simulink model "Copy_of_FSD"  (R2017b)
settings: Solver=FixedStepDiscrete  StartTime=0.0  StopTime=10.0  FixedStep=0.01  RelTol=1e-3  EnableMultiTasking=on
undefined symbols (not defined in the file): ASWTYPE_FALSE, ASWTYPE_TRUE, CcFSD_MSDOpenFltDelTi_ms, CcFSD_MSDOpenPackVolt_V, CcFSD_MSDOpenSumCellVolt_V, FSD_RUNTIME_MS
libraries: AIWAYS_Powertrain_BMS_lib x6

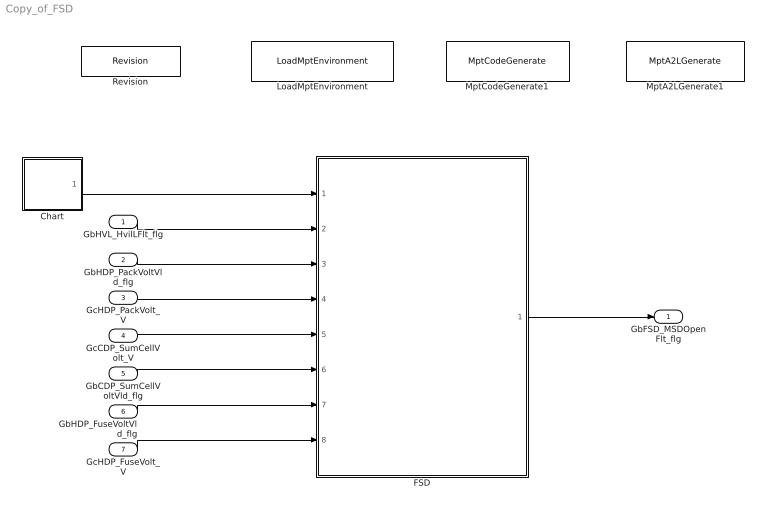
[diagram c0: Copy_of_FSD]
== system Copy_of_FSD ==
  GbHVL_HvilLFlt_flg : Inport
  GbHDP_PackVoltVld_flg : Inport  Port=2
  GcHDP_PackVolt_V : Inport  Port=3
  GcCDP_SumCellVolt_V : Inport  Port=4
  GbCDP_SumCellVoltVld_flg : Inport  Port=5
  GbHDP_FuseVoltVld_flg : Inport  Port=6
  GcHDP_FuseVolt_V : Inport  Port=7
  Chart : Stateflow chart  TreatAsAtomicUnit=on
  FSD : Subsystem
  LoadMptEnvironment : AIWAYS_Powertrain_BMS_lib/Config/LoadMptEnvironment  ProjectName=Comm  SuppierID=NewPlatformUAES
  MptA2LGenerate1 : AIWAYS_Powertrain_BMS_lib/Config/MptA2LGenerate  SystemSampleTime=-1
  MptCodeGenerate1 : AIWAYS_Powertrain_BMS_lib/Config/MptCodeGenerate  SystemSampleTime=-1
  Revision : AIWAYS_Powertrain_BMS_lib/Config/Revision  curVersion='M101C100'  newVersion='M101C100'
  GbFSD_MSDOpenFlt_flg : Outport
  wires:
  Chart/1(FSD_FuseDiag_100ms()) -> FSD/1(FSD_FuseDiag_100ms)
  GbHVL_HvilLFlt_flg/1 -> FSD/2(GbHVL_HvilLFlt_flg)
  GbHDP_PackVoltVld_flg/1 -> FSD/3(GbHDP_PackVoltVld_flg)
  GcHDP_PackVolt_V/1 -> FSD/4(GcHDP_PackVolt_V)
  GcCDP_SumCellVolt_V/1 -> FSD/5(GcCDP_SumCellVolt_V)
  GbCDP_SumCellVoltVld_flg/1 -> FSD/6(GbCDP_SumCellVoltVld_flg)
  FSD/1(GbFSD_MSDOpenFlt_flg) -> GbFSD_MSDOpenFlt_flg/1
  GbHDP_FuseVoltVld_flg/1 -> FSD/7(GbHDP_FuseVoltVld_flg)
  GcHDP_FuseVolt_V/1 -> FSD/8(GcHDP_FuseVolt_V)

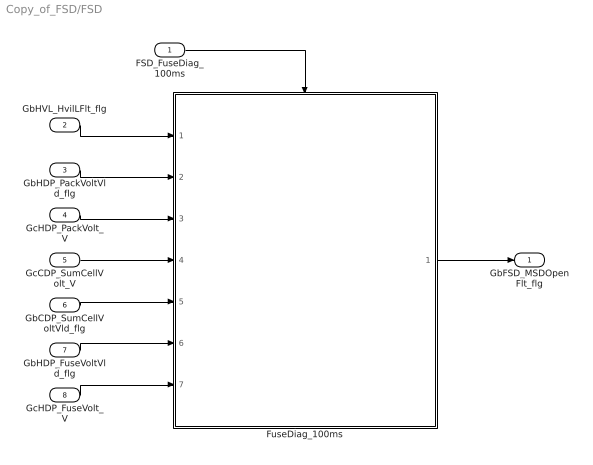
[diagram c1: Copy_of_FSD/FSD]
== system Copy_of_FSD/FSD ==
  FSD_FuseDiag_100ms : Inport
  GbHVL_HvilLFlt_flg : Inport  Port=2
  GbHDP_PackVoltVld_flg : Inport  Port=3
  GcHDP_PackVolt_V : Inport  Port=4
  GcCDP_SumCellVolt_V : Inport  Port=5
  GbCDP_SumCellVoltVld_flg : Inport  Port=6
  GbHDP_FuseVoltVld_flg : Inport  Port=7
  GcHDP_FuseVolt_V : Inport  Port=8
  FuseDiag_100ms : Subsystem
  GbFSD_MSDOpenFlt_flg : Outport
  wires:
  FSD_FuseDiag_100ms/1 -> FuseDiag_100ms/Trigger
  GbHDP_PackVoltVld_flg/1 -> FuseDiag_100ms/2(GbHDP_PackVoltVld_flg)
  GcHDP_PackVolt_V/1 -> FuseDiag_100ms/3(GcHDP_PackVolt_V)
  GbHVL_HvilLFlt_flg/1 -> FuseDiag_100ms/1(GbHVL_HvilLFlt_flg)
  GcCDP_SumCellVolt_V/1 -> FuseDiag_100ms/4(GcCDP_SumCellVolt_V)
  GbCDP_SumCellVoltVld_flg/1 -> FuseDiag_100ms/5(GbCDP_SumCellVoltVld_flg)
  FuseDiag_100ms/1(GbFSD_MSDOpenFlt_flg) -> GbFSD_MSDOpenFlt_flg/1
  GbHDP_FuseVoltVld_flg/1 -> FuseDiag_100ms/6(GbHDP_FuseVoltVld_flg)
  GcHDP_FuseVolt_V/1 -> FuseDiag_100ms/7(GcHDP_FuseVolt_V)

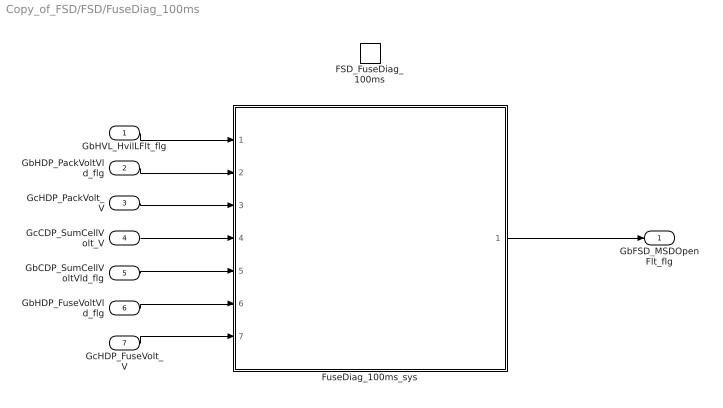
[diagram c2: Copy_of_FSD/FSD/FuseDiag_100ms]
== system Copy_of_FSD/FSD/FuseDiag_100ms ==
  GbHVL_HvilLFlt_flg : Inport
  GbHDP_PackVoltVld_flg : Inport  Port=2
  GcHDP_PackVolt_V : Inport  Port=3
  GcCDP_SumCellVolt_V : Inport  Port=4
  GbCDP_SumCellVoltVld_flg : Inport  Port=5
  GbHDP_FuseVoltVld_flg : Inport  Port=6
  GcHDP_FuseVolt_V : Inport  Port=7
  FSD_FuseDiag_100ms : TriggerPort  TriggerType=function-call  VariantControl=(inherit)
  FuseDiag_100ms_sys : Subsystem
  GbFSD_MSDOpenFlt_flg : Outport
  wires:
  GbHVL_HvilLFlt_flg/1 -> FuseDiag_100ms_sys/1(GbHVL_HvilLFlt_flg)
  GbHDP_PackVoltVld_flg/1 -> FuseDiag_100ms_sys/2(GbHDP_PackVoltVld_flg)
  GcHDP_PackVolt_V/1 -> FuseDiag_100ms_sys/3(GcHDP_PackVolt_V)
  GcCDP_SumCellVolt_V/1 -> FuseDiag_100ms_sys/4(GcCDP_SumCellVolt_V)
  GbCDP_SumCellVoltVld_flg/1 -> FuseDiag_100ms_sys/5(GbCDP_SumCellVoltVld_flg)
  FuseDiag_100ms_sys/1(GbFSD_MSDOpenFlt_flg) -> GbFSD_MSDOpenFlt_flg/1
  GbHDP_FuseVoltVld_flg/1 -> FuseDiag_100ms_sys/6(GbHDP_FuseVoltVld_flg)
  GcHDP_FuseVolt_V/1 -> FuseDiag_100ms_sys/7(GcHDP_FuseVolt_V)

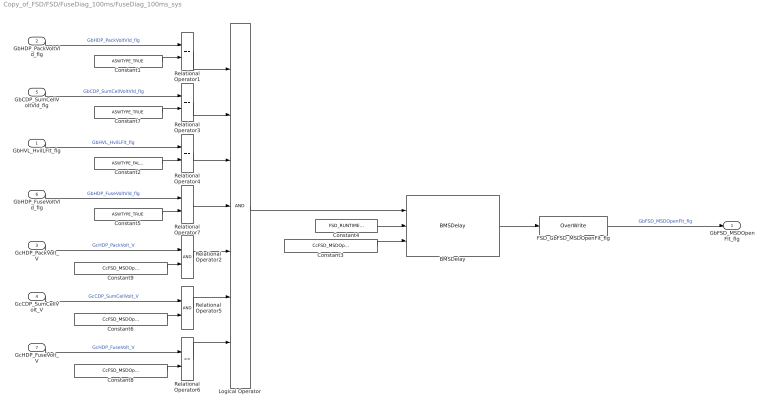
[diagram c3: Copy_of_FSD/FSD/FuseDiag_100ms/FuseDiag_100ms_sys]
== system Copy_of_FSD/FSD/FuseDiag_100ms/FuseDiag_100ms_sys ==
  GbHVL_HvilLFlt_flg : Inport
  GbHDP_PackVoltVld_flg : Inport  Port=2
  GcHDP_PackVolt_V : Inport  Port=3
  GcCDP_SumCellVolt_V : Inport  Port=4
  GbCDP_SumCellVoltVld_flg : Inport  Port=5
  GbHDP_FuseVoltVld_flg : Inport  Port=6
  GcHDP_FuseVolt_V : Inport  Port=7
  BMSDelay : AIWAYS_Powertrain_BMS_lib/Debounce & Delay/BMSDelay
  Constant1 : Constant  Value=ASWTYPE_TRUE
  Constant2 : Constant  Value=ASWTYPE_FALSE
  Constant3 : Constant  Value=CcFSD_MSDOpenFltDelTi_ms
  Constant4 : Constant  Value=FSD_RUNTIME_MS
  Constant5 : Constant  Value=ASWTYPE_TRUE
  Constant6 : Constant  Value=CcFSD_MSDOpenSumCellVolt_V
  Constant7 : Constant  Value=ASWTYPE_TRUE
  Constant8 : Constant  Value=CcFSD_MSDOpenPackVolt_V
  Constant9 : Constant  Value=CcFSD_MSDOpenSumCellVolt_V
  FSD_GbFSD_MSDOpenFlt_flg : AIWAYS_Powertrain_BMS_lib/Signals/OverWrite  OverWrite_Value=CbFSD_MSDOpenFltOvr_flg  OverWrite_flag=CbFSD_MSDOpenFltOvrSwt_flg
  Logical Operator : Logic  Inputs=7  AllPortsSameDT=off  OutDataTypeStr=boolean
  Relational Operator{1,3..4,7} (4 alike) : RelationalOperator  Operator===  OutDataTypeStr=boolean
  Relational Operator2 : RelationalOperator  OutDataTypeStr=boolean
  Relational Operator5 : RelationalOperator  OutDataTypeStr=boolean
  Relational Operator6 : RelationalOperator  Operator=<=  OutDataTypeStr=boolean
  GbFSD_MSDOpenFlt_flg : Outport
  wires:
  Constant1/1 -> Relational Operator1/2
  GbHDP_PackVoltVld_flg/1 -> Relational Operator1/1  "GbHDP_PackVoltVld_flg"
  Constant7/1 -> Relational Operator3/2
  GbCDP_SumCellVoltVld_flg/1 -> Relational Operator3/1  "GbCDP_SumCellVoltVld_flg"
  Constant2/1 -> Relational Operator4/2
  GbHVL_HvilLFlt_flg/1 -> Relational Operator4/1  "GbHVL_HvilLFlt_flg"
  GcHDP_PackVolt_V/1 -> Relational Operator2/1  "GcHDP_PackVolt_V"
  GcCDP_SumCellVolt_V/1 -> Relational Operator5/1  "GcCDP_SumCellVolt_V"
  Constant3/1 -> BMSDelay/3
  Logical Operator/1 -> BMSDelay/1
  Constant4/1 -> BMSDelay/2
  Relational Operator1/1 -> Logical Operator/1
  Relational Operator3/1 -> Logical Operator/2
  Relational Operator4/1 -> Logical Operator/3
  Relational Operator2/1 -> Logical Operator/5
  Relational Operator5/1 -> Logical Operator/6
  BMSDelay/1 -> FSD_GbFSD_MSDOpenFlt_flg/1
  Constant9/1 -> Relational Operator2/2
  Constant6/1 -> Relational Operator5/2
  FSD_GbFSD_MSDOpenFlt_flg/1 -> GbFSD_MSDOpenFlt_flg/1  "GbFSD_MSDOpenFlt_flg"
  Constant8/1 -> Relational Operator6/2
  Constant5/1 -> Relational Operator7/2
  GbHDP_FuseVoltVld_flg/1 -> Relational Operator7/1  "GbHDP_FuseVoltVld_flg"
  GcHDP_FuseVolt_V/1 -> Relational Operator6/1  "GcHDP_FuseVolt_V"
  Relational Operator6/1 -> Logical Operator/7
  Relational Operator7/1 -> Logical Operator/4

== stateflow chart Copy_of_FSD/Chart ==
  state OS
    (default) -> (junction 1) : {i = uint8(0);}
    OS -> (junction 1)
    (junction 1) -> (junction 3)
    (junction 3) -> (junction 9) : [i>uint8(9)]
    (junction 9) -> (junction 7) : { FSD_FuseDiag_100ms; i = uint8(0); }
    (junction 3) -> (junction 7) : {i = i + 1;}
  data: i local uint8
  events: output FUNCTION_CALL_EVENT
